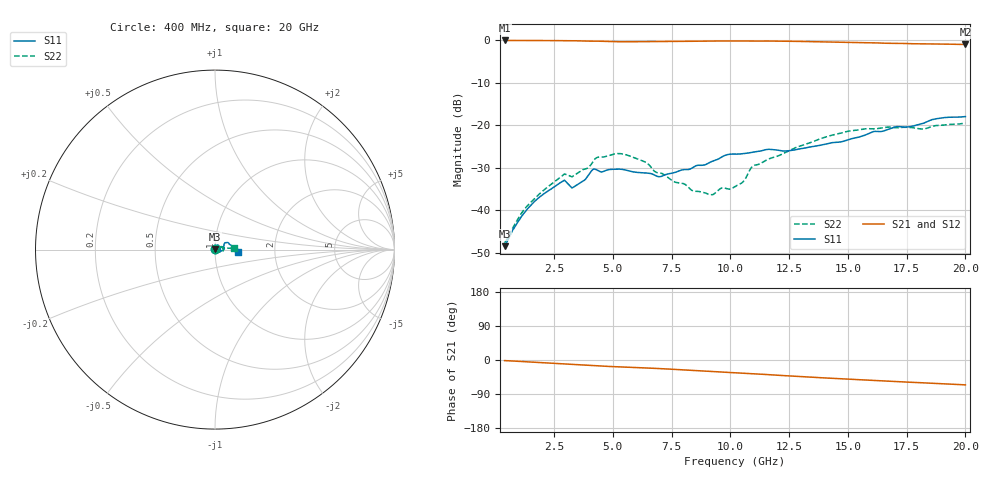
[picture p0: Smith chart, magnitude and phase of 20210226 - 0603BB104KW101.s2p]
!Keysight Technologies,N5227A,US56070614,A.10.47.06
!Date: Tuesday, May 21, 2019 12:49:52
!Correction: S11(Full 2 Port(1,2))
!S21(Full 2 Port(1,2))
!S12(Full 2 Port(1,2))
!S22(Full 2 Port(1,2))
!S2P File: Measurements: S11, S21, S12, S22:
# Hz S  dB  R 50
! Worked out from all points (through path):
!   801 points, 400 MHz to 20 GHz, reference 50 ohm
!   highest |S21| = -0.01 dB at 400 MHz (marker M1); lowest = -1.0 dB at 20 GHz (marker M2)
!   group delay of S21, straight-line fit = 9.17 ps
!   lowest |S11| = -48.4 dB at 400 MHz (marker M3), VSWR 1.01, Z = 50.1 + j0.36 ohm
!   |S11| at or under -10 dB: start of sweep to end of sweep
!   |S22| runs from -47.6 to -19.4 dB; largest |S21 - S12| = 0.00073
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4e8  -48.42 70.9  -0.01 -1.6  -0.01 -1.6  -47.64 69.5
1.184e9  -40.93 82.3  -0.02 -4.2  -0.01 -4.2  -40.16 66.4
1.87e9  -36.94 86.1  -0.03 -6.7  -0.02 -6.7  -36.18 59.6
2.8745e9  -33.12 85.1  -0.06 -10.4  -0.05 -10.4  -31.77 49.4
3.291e9  -34.65 74.6  -0.08 -11.9  -0.07 -11.9  -32.00 38.1
3.683e9  -33.25 69.0  -0.11 -13.3  -0.11 -13.3  -30.55 32.3
4.1975e9  -30.27 52.0  -0.17 -14.9  -0.17 -14.9  -28.19 29.1
5.2755e9  -30.29 10.7  -0.32 -18.0  -0.31 -18.0  -26.63 -0.1
6.3535e9  -31.17 -18.3  -0.27 -20.7  -0.26 -20.7  -28.55 -20.6
6.9415e9  -32.06 -25.8  -0.25 -22.5  -0.25 -22.5  -31.18 -21.6
8.4115e9  -29.89 -16.1  -0.20 -27.3  -0.20 -27.3  -35.41 -11.0
9.122e9  -28.72 -10.7  -0.16 -29.7  -0.15 -29.7  -36.31 3.7
9.6365e9  -27.44 -6.8  -0.13 -31.5  -0.13 -31.5  -34.73 14.6
1.02e10  -26.75 -8.1  -0.14 -33.7  -0.13 -33.7  -34.40 24.2
1.0543e10  -26.63 -5.2  -0.15 -34.9  -0.15 -34.9  -33.28 32.2
1.0984e10  -26.25 -0.5  -0.17 -36.3  -0.17 -36.3  -29.49 28.9
1.3483e10  -25.00 27.6  -0.29 -45.5  -0.29 -45.5  -23.89 8.2
1.5002e10  -23.39 34.4  -0.46 -50.5  -0.46 -50.5  -21.38 4.9
1.67415e10  -20.90 17.2  -0.68 -56.0  -0.68 -56.0  -20.39 5.4
1.82115e10  -19.49 -2.7  -0.81 -60.2  -0.81 -60.2  -20.86 6.7
1.8873e10  -18.34 -6.5  -0.85 -62.2  -0.85 -62.2  -19.99 6.0
2e10  -17.92 -7.2  -0.96 -65.6  -0.96 -65.6  -19.44 3.7
